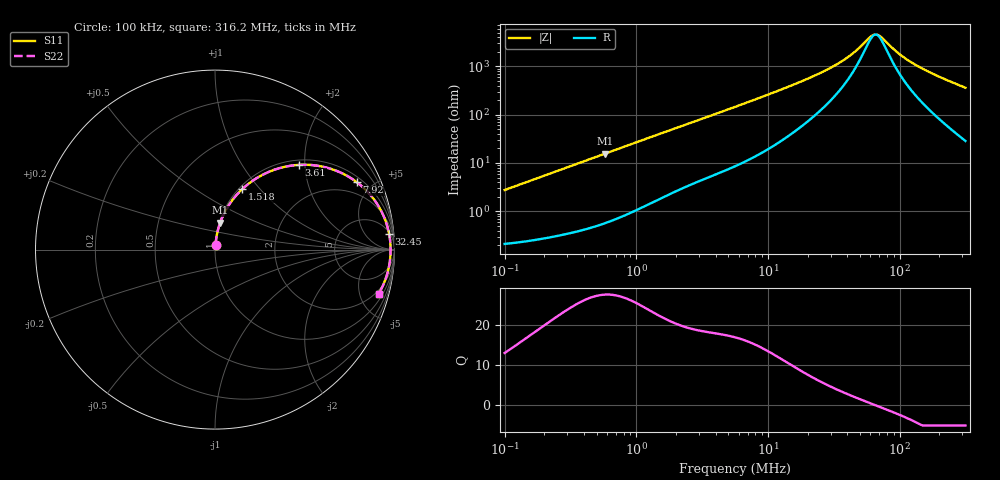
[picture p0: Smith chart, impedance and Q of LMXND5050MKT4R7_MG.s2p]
! LMXND5050MKT4R7_MG  S-PARAMETER MODEL  ( General Type )
! Model Generated by TAIYO YUDEN Corporation (http://www.ty-top.com)
! Version 1.0
! TAIYO YUDEN Control No. 191023NI43SB-FBB
! Copyright(c) 2019 TAIYO YUDEN CO.,LTD. All Rights Reserved.
! Product Description (link to TY-COMPAS)
! https://ds.yuden.co.jp/TYCOMPAS/or/detail?pn=LMXND5050MKT4R7MMG&u=M
! Products Name : Inductors
! Characteristics :
!  Inductance : 4.7 uH , SRF(min) : 40 MHz , DC Resistance(max) : 0.216 Ohm
!  Rated Current : Saturation :2200 mA , Temp Rise : 1400 mA
!  Case Size : 4.9 x 4.9 / 0.193 x 0.193 [mm/inch] , Thickness : 1.2 / 0.047 [mm/inch]
!  (Conditions: Temperature = 25 degC , DC Bias Current/Voltage = 0A / 0V)
! External Node Assignments :
!  1  o---GGG---o  2
! GND o---------o GND
! Frequency Range : 0.1MHz  -  316.199832MHz  [ 402 STEP ]
# MHz S RI R 50
! Freq[MHz].  S11 Real  S11 Imag  S21 Real  S21 Imag  S12 Real  S12 Imag  S22 Real  S22 Imag
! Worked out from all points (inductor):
!   401 points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, 100 kHz to 316.2 MHz, reference 50 ohm
!   read as one part in series: L = 4.37 uH near 104.1 kHz
!   highest Q = 27.5 at 577.1 kHz (marker M1), where L = 4.3 uH
!   self-resonance near 65.87 MHz
!   S11 on the Smith chart (normalised r, x): 100 kHz: 1.00, +0.06; 1.518 MHz: 1.04, +0.81; 3.61 MHz: 1.10, +1.87; 7.92 MHz: 1.27, +4.08; 32.45 MHz: 6, +20; 316.2 MHz: 1.57, -7.21
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0.1  0.00287 0.0274  0.9971 -0.0274  0.9971 -0.0274  0.00287 0.0274
0.385695  0.0147 0.1027  0.9853 -0.1027  0.9853 -0.1027  0.0147 0.1027
0.577087  0.029 0.1505  0.971 -0.1505  0.971 -0.1505  0.029 0.1505
0.974404  0.0722 0.2401  0.9278 -0.2401  0.9278 -0.2401  0.0722 0.2401
1.487603  0.1464 0.3318  0.8536 -0.3318  0.8536 -0.3318  0.1464 0.3318
1.517879  0.1512 0.3363  0.8488 -0.3363  0.8488 -0.3363  0.1512 0.3363
2.271094  0.2731 0.4208  0.7269 -0.4208  0.7269 -0.4208  0.2731 0.4208
3.609798  0.4689 0.4722  0.5311 -0.4722  0.5311 -0.4722  0.4689 0.4722
5.623165  0.6679 0.4423  0.3321 -0.4423  0.3321 -0.4423  0.6679 0.4423
7.920073  0.7915 0.3746  0.2085 -0.3746  0.2085 -0.3746  0.7915 0.3746
12.58859  0.897 0.2637  0.103 -0.2637  0.103 -0.2637  0.897 0.2637
21.68824  0.9533 0.1512  0.0467 -0.1512  0.0467 -0.1512  0.9533 0.1512
32.45058  0.9702 0.0875  0.0298 -0.0875  0.0298 -0.0875  0.9702 0.0875
43.02502  0.9758 0.0503  0.0242 -0.0503  0.0242 -0.0503  0.9758 0.0503
59.39086  0.9784 0.0119  0.0216 -0.0119  0.0216 -0.0119  0.9784 0.0119
63.09128  0.9785 0.00495  0.0215 -0.00495  0.0215 -0.00495  0.9785 0.00495
69.77805  0.9785 -0.00663  0.0215 0.00663  0.0215 0.00663  0.9785 -0.00663
83.65039  0.9778 -0.0277  0.0222 0.0277  0.0222 0.0277  0.9778 -0.0277
104.4039  0.9756 -0.0547  0.0244 0.0547  0.0244 0.0547  0.9756 -0.0547
138.4253  0.9698 -0.0926  0.0302 0.0926  0.0302 0.0926  0.9698 -0.0926
202.9849  0.9537 -0.1544  0.0463 0.1544  0.0463 0.1544  0.9537 -0.1544
316.1998  0.9123 -0.246  0.0877 0.246  0.0877 0.246  0.9123 -0.246
